TYPE Alm_EventClass :
(
    NoAlarm                  :=0,(*无警报*)
    Message_1      :=1,(*信息*)
    Event_2            :=2,(*事件*)
    non_3                        :=3,(*暂无*)
    non_4                       :=4,(*暂无*)
    non_5                         :=5,(*暂无*)
    Alarm_6          :=6,(*不停机警报*)
    Stop_7                :=7(*停机警报*)
);
END_TYPE
